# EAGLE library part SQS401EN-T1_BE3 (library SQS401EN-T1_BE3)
MOSFET P-CHANNEL 40V (D-S) Source: Datasheet
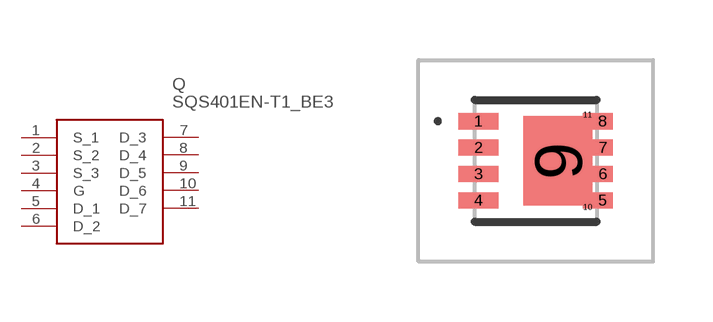
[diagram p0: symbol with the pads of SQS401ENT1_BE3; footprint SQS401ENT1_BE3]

Designator prefix Q

## SQS401EN-T1_BE3 (Arrow_Part_Number: SQS401EN-T1_BE3; Arrow_Price-Stock: https://www.arrow.com/en/products/sqs401en-t1-be3/vishay?region=nac; Description: MOSFET P-CHANNEL 40V (D-S); Height: 1.12mm; Manufacturer_Name: Vishay; Manufacturer_Part_Number: SQS401EN-T1_BE3; Mouser_Part_Number: 78-SQS401EN-T1_BE3; Mouser_Price-Stock: https://www.mouser.co.uk/ProductDetail/Vishay-Siliconix/SQS401EN-T1_BE3?qs=TiOZkKH1s2Te3TfnWUAn6g%3D%3D)  [SQS401ENT1_BE3]
1  S_1
2  S_2
3  S_3
4  G
5  D_1
6  D_2
7  D_3
8  D_4
9  D_5
10  D_6
11  D_7

## Footprint SQS401ENT1_BE3 (pad centres in mm)
SQS401EN-T1_BE3-3
smd 0.99 x 0.405: 1 -1.435,0.99; 2 -1.435,0.33; 3 -1.435,-0.33; 4 -1.435,-0.99
smd 0.51 x 0.405: 5 1.675,-0.99; 6 1.675,-0.33; 7 1.675,0.33; 8 1.675,0.99
smd 1.725 x 2.235: 9 0.557,0
smd 0.25 x 0.077: 10 1.295,-1.156; 11 1.295,1.156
